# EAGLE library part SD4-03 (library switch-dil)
DIL/CODE SWITCH
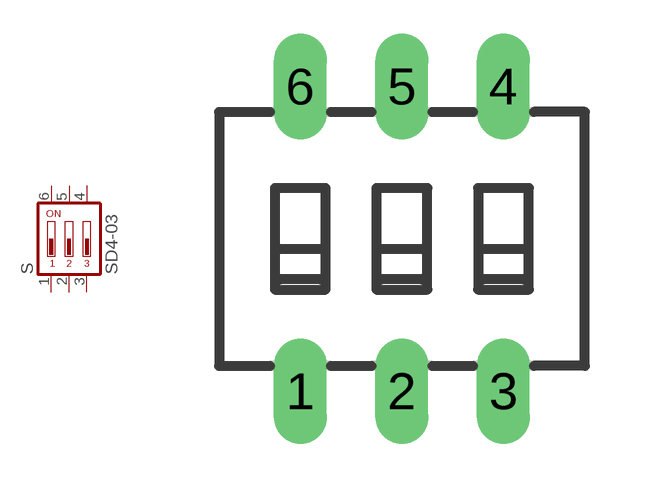
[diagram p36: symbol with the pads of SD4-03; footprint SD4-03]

Designator prefix S

## SD4-03 (OC_FARNELL: unknown; OC_NEWARK: unknown)  [SD4-03]
1  1  pas
2  2  pas
3  3  pas
4  4  pas
5  5  pas
6  6  pas

## Footprint SD4-03 (pad centres in mm)
DIL/CODE SWITCH Mors
drill 0.813 long: 1 -2.54,-3.81; 2 0,-3.81; 3 2.54,-3.81; 4 2.54,3.81; 5 0,3.81; 6 -2.54,3.81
